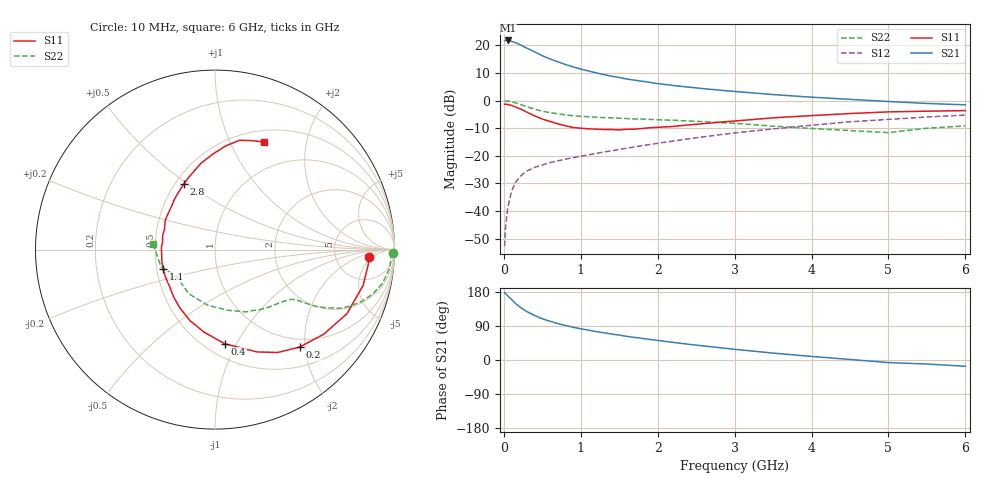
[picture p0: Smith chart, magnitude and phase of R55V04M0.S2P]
! SIEMENS Small Signal Semiconductors
! BFR183
! Si NPN RF Bipolar Junction Transistor in SOT23
! VCE = 5 V  IC = 4 mA
! Common Emitter S-Parameters:  May  1996
# GHz  S  MA  R  50
!  f  S11  S21  S12  S22
! GHz  MAG  ANG  MAG  ANG  MAG  ANG  MAG  ANG
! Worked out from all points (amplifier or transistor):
!   36 points, 10 MHz to 6 GHz, reference 50 ohm
!   highest |S21| = 21.8 dB at 50 MHz (marker M1)
!   |S21| within 3 dB of that: start of sweep to 314.1 MHz
!   unconditionally stable (mu >= 1): 1.15 GHz to 2.706 GHz
!   at 250 MHz: K = 0.36, MSG = 23.1 dB, |S12| = -26.5 dB
!   at 1.4 GHz: K = 1.05, MAG = 12.1 dB, |S12| = -18.2 dB
!   at 6 GHz: K = 0.88, MSG = 1.9 dB, |S12| = -5.2 dB
!   S11 on the Smith chart (normalised r, x): 10 MHz: 12, -4; 200 MHz: 0.84, -1.89; 400 MHz: 0.62, -0.90; 1.1 GHz: 0.54, -0.13; 2.8 GHz: 0.55, +0.49; 6 GHz: 0.64, +1.36
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0.01  0.8603 -2.7  12.24 178.0  0.0023 90.3  0.9917 -1.2
0.02  0.8582 -5.4  12.2 175.6  0.0047 82.2  0.9805 -2.2
0.05  0.8493 -13.5  12.3 169.4  0.0114 82.6  0.9803 -5.8
0.1  0.8175 -25.9  11.84 159.7  0.0227 77.4  0.9526 -11.3
0.15  0.7675 -37.9  11.23 149.4  0.0327 70.5  0.9115 -15.9
0.2  0.7193 -49.0  10.54 141.2  0.0401 66.4  0.8631 -19.7
0.25  0.6711 -58.7  9.651 134.1  0.0472 62.2  0.8162 -22.7
0.3  0.6162 -67.7  8.893 127.6  0.0529 59.7  0.776 -24.9
0.4  0.528 -84.0  7.647 117.5  0.0617 55.8  0.6993 -27.7
0.5  0.4638 -97.6  6.516 108.8  0.0681 53.9  0.6423 -29.4
0.6  0.4187 -109.6  5.684 102.2  0.0752 53.0  0.6056 -30.2
0.7  0.3797 -121.0  5.052 96.3  0.0809 52.9  0.5771 -30.8
0.9  0.3258 -141.0  4.082 86.4  0.0925 53.7  0.5324 -31.7
1.1  0.3081 -159.4  3.441 78.8  0.1041 54.9  0.5081 -33.2
1.4  0.2988 177.8  2.763 68.6  0.123 56.4  0.4867 -35.9
1.6  0.3022 165.1  2.46 62.3  0.1373 56.6  0.4723 -38.0
2.2  0.3402 135.9  1.879 46.5  0.1849 56.6  0.4403 -46.7
2.8  0.4061 115.2  1.548 32.7  0.2397 53.3  0.3986 -58.5
3.5  0.487 99.3  1.286 18.2  0.3065 46.9  0.3448 -78.3
4.5  0.5823 83.9  1.054 1.4  0.413 35.4  0.286 -120.5
5.5  0.6427 70.8  0.887 -10.6  0.5046 22.7  0.3157 -162.2
6  0.6589 65.3  0.838 -16.5  0.5473 14.3  0.3475 174.4
